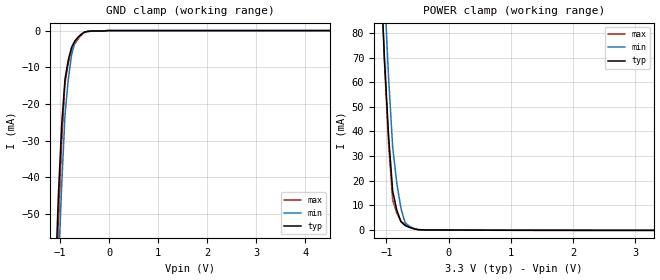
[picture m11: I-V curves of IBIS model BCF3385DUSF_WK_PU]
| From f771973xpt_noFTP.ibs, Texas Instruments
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|BCF3385DUSF_WK_PD; WEAK_PULLDOWN_ON
|   Model Cell  BCF3385DUSF_WK_PU
| BCF3385DUSF_WK_PU
[Model]   BCF3385DUSF_WK_PU
Model_type   Input
Polarity   Non-Inverting
Vinl =  0.8
Vinh =  2
C_comp   1.190763p   1.060544p   1.317111p
[Model Spec]
Vinl   0.8   0.8   0.8
Vinh   2   2   2
[Temperature Range]   25   155   -40
[Voltage Range]   3.3   2.97   3.63
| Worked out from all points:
|   GND clamp passes 1 mA (typ) near -0.57 V on its own axis
|   POWER clamp passes 1 mA (typ) near -0.62 V on its own axis
| Nom Voltages:
|   VDD=1.2, VDDS=3.3, VSS=0
| Min Voltages:
|   VDD=1.08, VDDS=2.97, VSS=0
| Max Voltages:
|   VDD=1.32, VDDS=3.63, VSS=0
[POWER_clamp]
|   voltage   I(typ)   I(min)   I(max)
-3.3V     1.919A     2.431A     2.07A
-1.1V     109.6mA    140.7mA    112.7mA
-1.033V   69.93mA    97.96mA    68.79mA
-966.7mV  38.67mA    62.26mA    35.25mA
-900mV    15.77mA    33.62mA    12.07mA
-833.3mV  8.066mA    18.98mA    6.794mA
-766.7mV  3.416mA    8.771mA    3.541mA
-700mV    1.823mA    2.98mA     2.308mA
-566.7mV  559.2uA    662uA      706.9uA
-500mV    180.3uA    246.1uA    210.5uA
-366.7mV  40uA       41.55uA    52.52uA
3.3V      -108.8uA   -62.53uA   -174uA
[GND_clamp]
|   voltage   I(typ)   I(min)   I(max)
-3.3V     -1.48A     -1.41A     -2.186A
-1.1V     -69.74mA   -89.96mA   -82.84mA
-1.033V   -44.48mA   -64.24mA   -52.89mA
-966.7mV  -25.64mA   -41.94mA   -30.09mA
-900mV    -13.23mA   -23.07mA   -14.44mA
-833.3mV  -8.038mA   -13.34mA   -8.967mA
-766.7mV  -4.575mA   -6.694mA   -5.352mA
-700mV    -2.842mA   -3.12mA    -3.602mA
-566.7mV  -977.9uA   -997uA     -1.251mA
-500mV    -370.6uA   -431uA     -470.7uA
-33.33mV  0A         0A         0A
6.6V      0A         0A         0A
